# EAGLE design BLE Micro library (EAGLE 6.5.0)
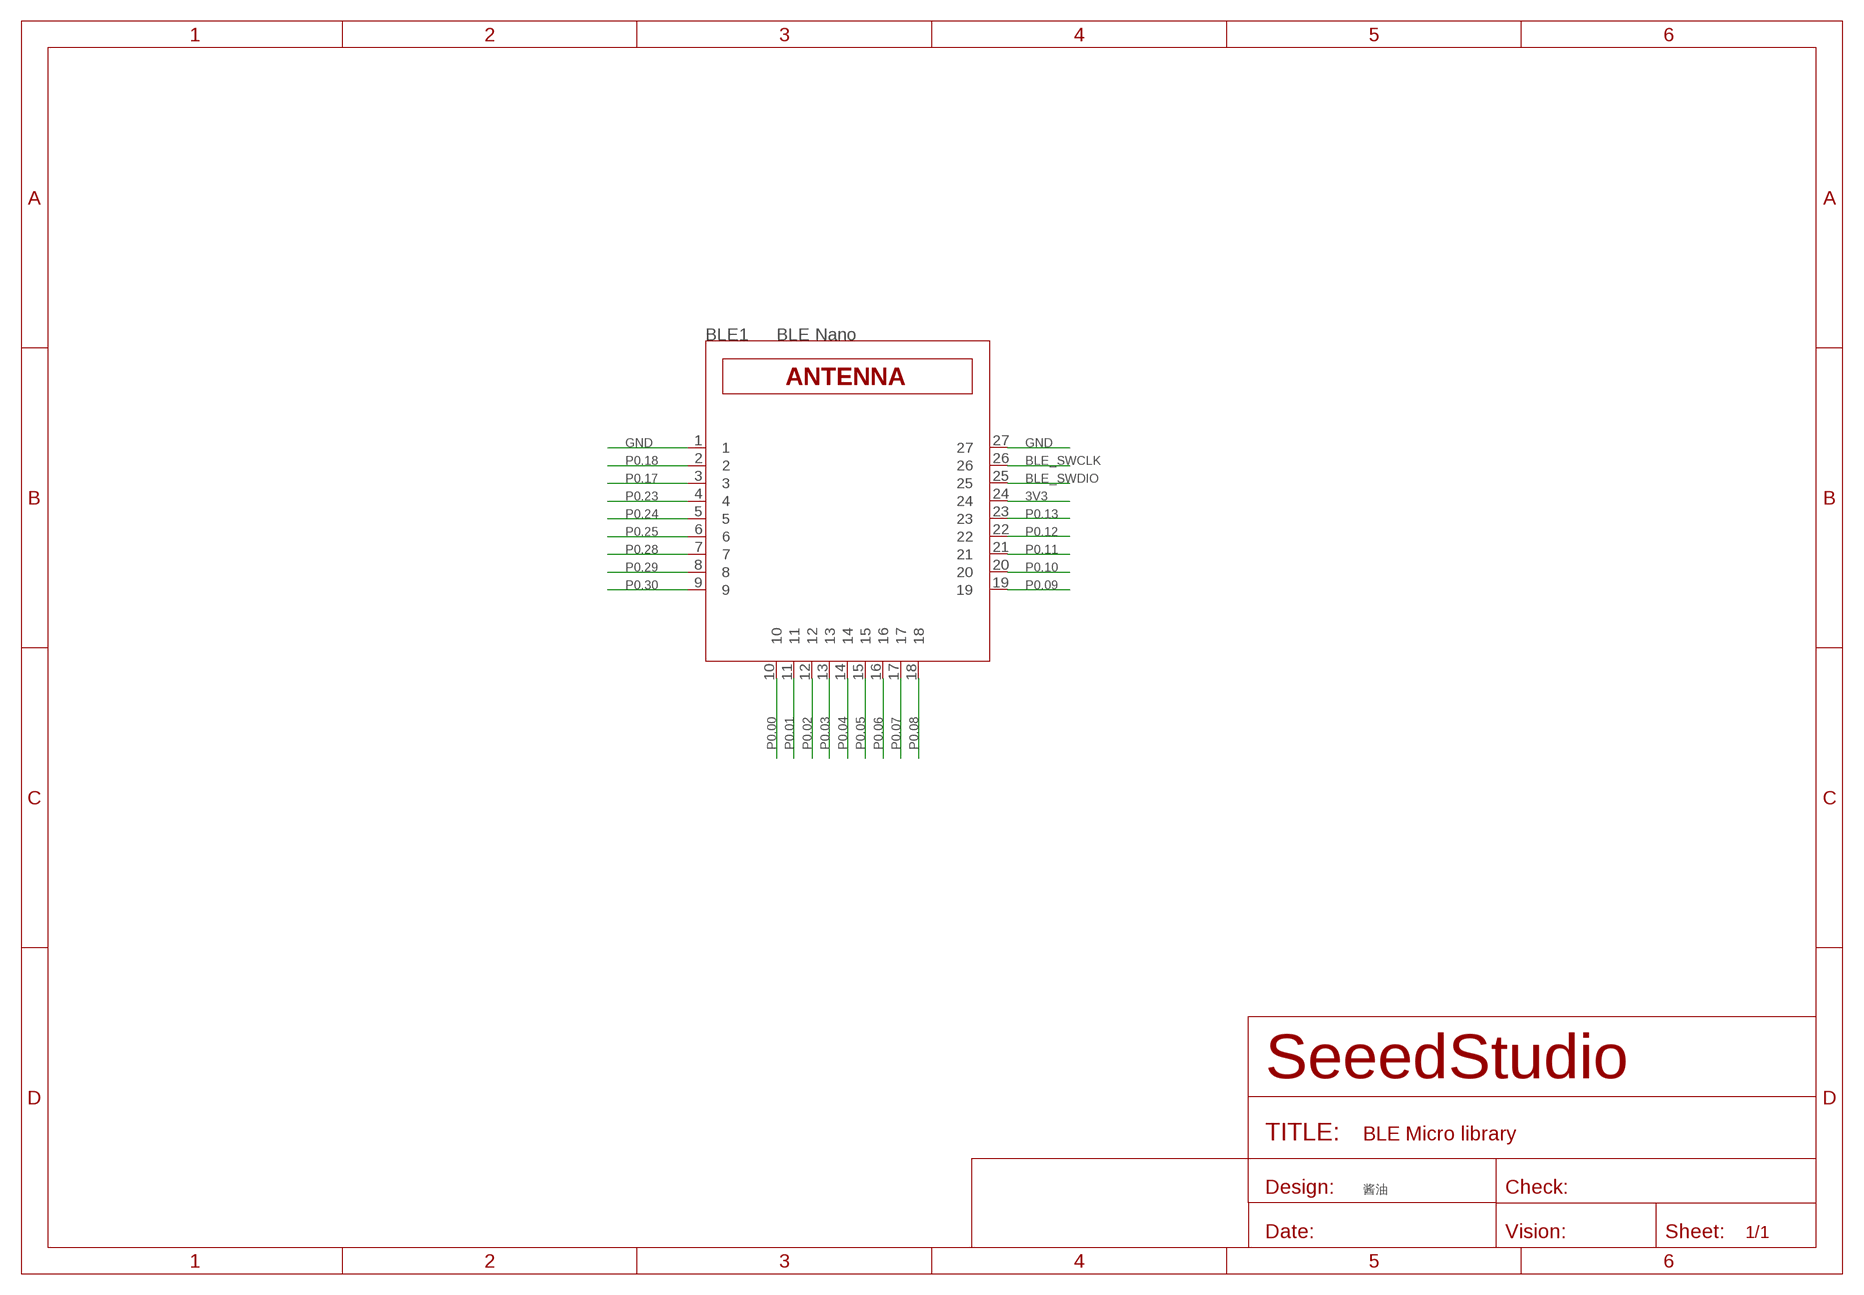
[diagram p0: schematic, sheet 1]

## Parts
BLE1  BLE Nano  SEEED_BLE_MODULE_001'PAD'  [SEEED_BLE_MODULE_PAD]

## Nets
3V3: BLE1.24
BLE_SWCLK: BLE1.26
BLE_SWDIO: BLE1.25
GND: BLE1.1 BLE1.27
P0.00: BLE1.10
P0.01: BLE1.11
P0.02: BLE1.12
P0.03: BLE1.13
P0.04: BLE1.14
P0.05: BLE1.15
P0.06: BLE1.16
P0.07: BLE1.17
P0.08: BLE1.18
P0.09: BLE1.19
P0.10: BLE1.20
P0.11: BLE1.21
P0.12: BLE1.22
P0.13: BLE1.23
P0.17: BLE1.3
P0.18: BLE1.2
P0.23: BLE1.4
P0.24: BLE1.5
P0.25: BLE1.6
P0.28: BLE1.7
P0.29: BLE1.8
P0.30: BLE1.9

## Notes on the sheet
- 酱油

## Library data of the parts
BLE1 = AMLib:SEEED_BLE_MODULE_001

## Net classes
0 default: width 0.102 mm, drill 0.203 mm, clearance 0.102 mm

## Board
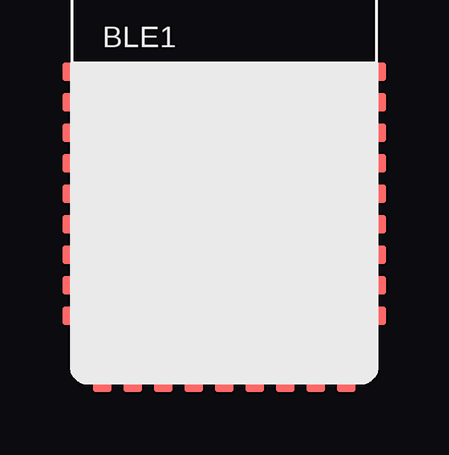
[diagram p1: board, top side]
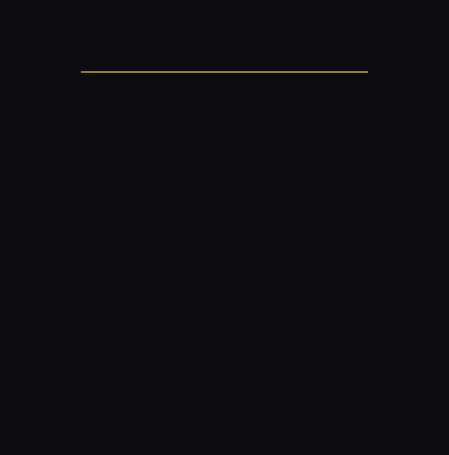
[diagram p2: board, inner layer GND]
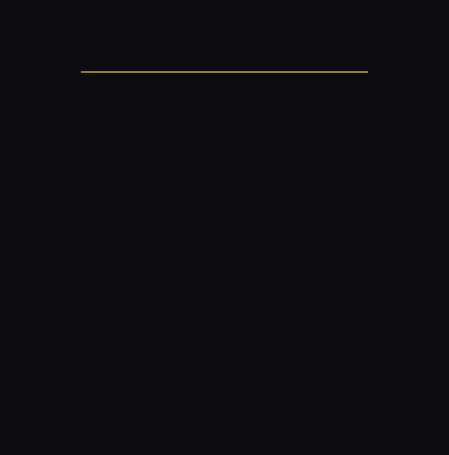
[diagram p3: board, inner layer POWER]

No outline drawn. Coordinates in mm, seen from the top.
Copper layers (1*2*15*16): Top 0.035mm / dielectric 0.2mm / GND 0.0175mm / dielectric 0.3mm / POWER 0.0175mm / dielectric 0.2mm / Bottom 0.035mm
Design rules "default *": minimum track width 6mil, minimum drill 12mil, track to track 6mil, track to pad 6mil, pad to pad 6mil, via to via 6mil, smd to smd 0mil, copper to edge 6mil, drill to drill 10mil, minimum pad ring 6mil, minimum via ring 6mil, stop-mask expansion 2mil, vias tented up to drill 25mil, thermal gap 10mil
tRestrict: area -1.3,4.3 to 3.7,9.3; area -0.3,9.4 to 0.1,10.2

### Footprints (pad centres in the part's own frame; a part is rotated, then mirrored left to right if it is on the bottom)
SEEED_BLE_MODULE_PAD = smd 1.524 x 0.762: 1 -5.969,12.954; 2 -5.969,11.684; 3 -5.969,10.414; 4 -5.969,9.144; 5 -5.969,7.874; 6 -5.969,6.604; 7 -5.969,5.334; 8 -5.969,4.064; 9 -5.969,2.794; 19 5.969,2.794; 20 5.969,4.064; 21 5.969,5.334; 22 5.969,6.604; 23 5.969,7.874; 24 5.969,9.144; 25 5.969,10.414; 26 5.969,11.684; 27 5.969,12.954 | smd 0.762 x 1.524: 10 -5.08,0.381; 11 -3.81,0.381; 12 -2.54,0.381; 13 -1.27,0.381; 14 0,0.381; 15 1.27,0.381; 16 2.54,0.381; 17 3.81,0.381; 18 5.08,0.381

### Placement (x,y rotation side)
BLE1  19.43,-0.13 0 top

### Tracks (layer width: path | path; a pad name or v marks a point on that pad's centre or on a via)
GND  (1 unrouted)
  pour GND (isolate 0.203, rank 5): -6.1,13.21 6.1,13.21 6.1,0.13 -6.1,0.13
VDD
  pour POWER (isolate 0.203): -6.1,13.21 6.1,13.21 6.1,0.13 -6.1,0.13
